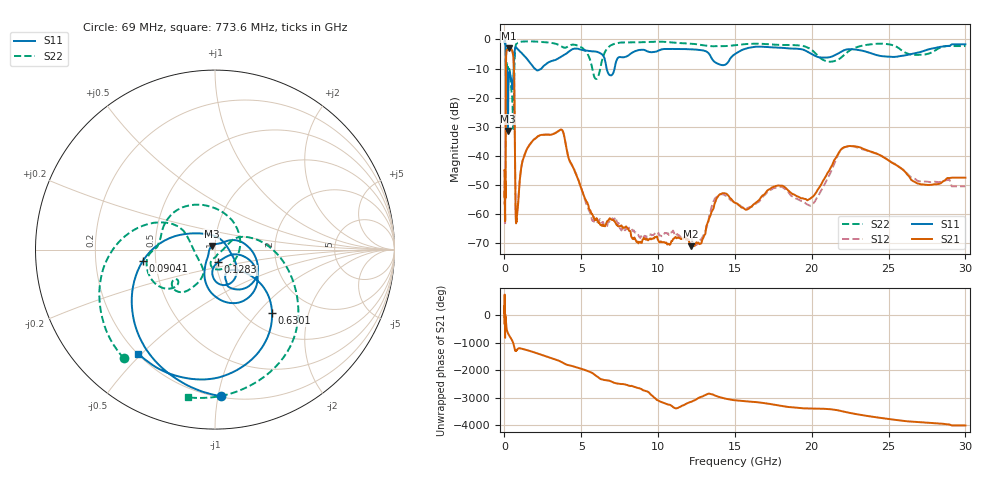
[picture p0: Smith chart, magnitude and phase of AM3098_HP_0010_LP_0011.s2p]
! Date/Time: Thu, Feb 28, 2019 8:32 AM
! Network Analyzer: Agilent Technologies E8364B Rev: A.07.50.67
! Sweep from 0.010 to 30.000 GHz, 1601 Points, Sweep Type: LOG
! Power Supply: 5.023 V, 0.002 A
# Hz S DB R 50
!freq MagS11 AngS11 MagS21 AngS21 MagS12 AngS12 MagS22 AngS22
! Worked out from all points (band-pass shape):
!   1601 points, 10 MHz to 30 GHz, reference 50 ohm
!   highest |S21| = -3.04 dB at 266.5 MHz (marker M1); lowest = -70.9 dB at 12.13 GHz (marker M2)
!   |S21| within 3 dB of the highest: 106.3 MHz to 576.7 MHz (470.3 MHz wide, 138 % of centre)
!   lowest |S11| = -31.4 dB at 227 MHz (marker M3), VSWR 1.06, Z = 48.2 + j1.93 ohm
!   |S11| at or under -10 dB: 175.4 MHz to 598.3 MHz (422.9 MHz wide, 109 % of centre); 1.975 GHz to 2.399 GHz (423.7 MHz wide, 19.4 % of centre); 6.649 GHz to 7.165 GHz (516.5 MHz wide, 7.48 % of centre)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
!   |S22| runs from -30.7 to -0.6 dB; largest |S21 - S12| = 0.011
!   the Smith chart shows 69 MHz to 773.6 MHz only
!   S11 on the Smith chart (normalised r, x): 69 MHz: 0.21, -1.02; 90.41 MHz: 0.43, -0.06; 128.3 MHz: 1.02, -0.15; 630.1 MHz: 1.31, -1.20; 773.6 MHz: 0.20, -0.49
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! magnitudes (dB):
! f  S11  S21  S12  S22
! 10 MHz  -0.4  -44.9  -44.9  -0.6
! 38.04 MHz  -0.5  -61.7  -61.5  -0.9
! 69 MHz  -1.8  -53.4  -51.7  -2.0
! 90.41 MHz  -7.9  -19.7  -19.6  -9.3
! 128.3 MHz  -22.8  -4.1  -4.1  -11.1
! 144.7 MHz  -13.8  -3.7  -3.6  -10.4
! 186.8 MHz  -11.5  -3.5  -3.5  -8.2
! 227 MHz  -31.4  -3.1  -3.1  -9.8
! 266.5 MHz  -14.8  -3.0  -3.0  -10.2
! 550.5 MHz  -15.9  -5.0  -4.9  -27.2
! 630.1 MHz  -6.4  -12.8  -12.7  -13.1
! 721.3 MHz  -2.7  -57.9  -57.1  -2.3
! 773.6 MHz  -2.8  -62.3  -61.6  -1.5
! 2.084 GHz  -10.5  -33.7  -33.6  -0.7
! 3.723 GHz  -5.8  -31.0  -31.0  -2.4
! 5.959 GHz  -4.2  -61.9  -62.8  -13.6
! 7.926 GHz  -5.9  -64.2  -65.1  -1.0
! 12.13 GHz  -3.4  -70.9  -67.7  -1.5
! 14.09 GHz  -8.7  -53.1  -53.2  -2.3
! 19.9 GHz  -4.7  -54.6  -57.1  -3.3
! 22.67 GHz  -3.4  -36.6  -36.6  -3.2
! 30 GHz  -1.7  -47.4  -50.4  -2.3
